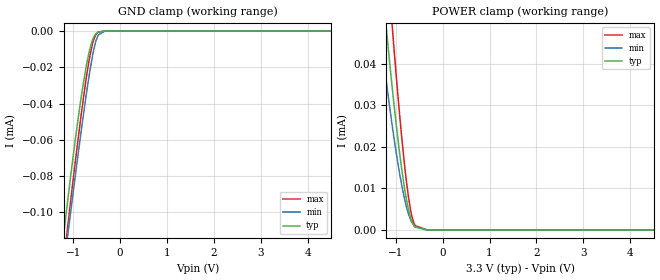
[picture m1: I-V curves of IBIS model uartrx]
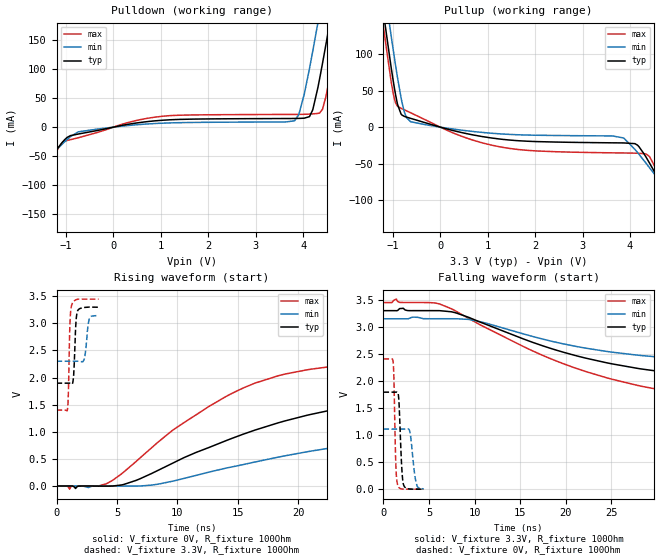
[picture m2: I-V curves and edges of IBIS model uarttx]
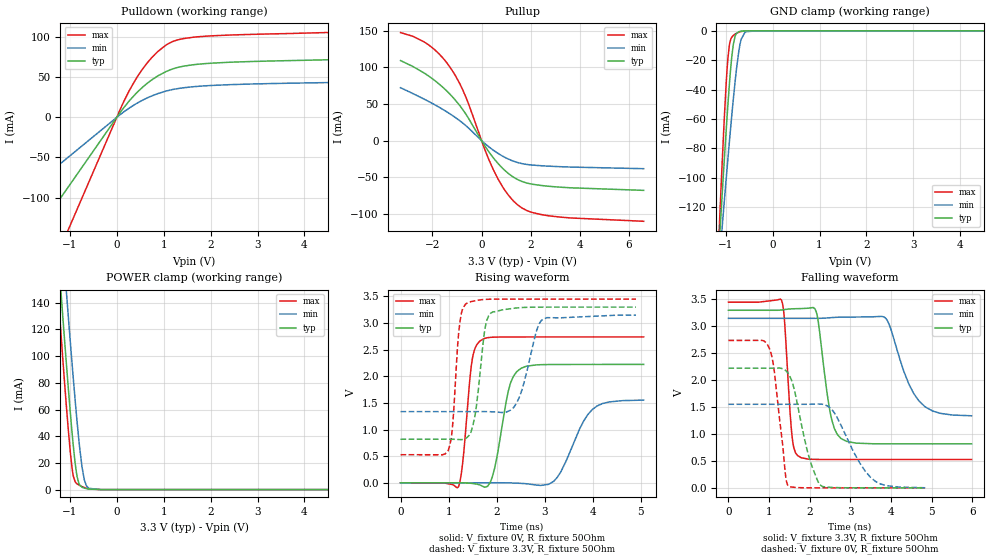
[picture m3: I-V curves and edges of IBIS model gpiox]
|Texas Instruments Incorporated
| NA
| Marketing part#   Digital Voltage Range   Package-type   #pins
| TPS65982ZQZ   3.15V-3.45V   BGA   96
[IBIS Ver]   4.1
[File name]   tps65982.ibs
[File Rev]   1.1
[Date]   8/31/2016
[Source]
| Texas Instruments Incorporated.
| Analog-eLab Design Center, HPA
| 12500 TI Blvd
| Dallas, TX -75243
[Notes]   Revision History:
| Rev 1.1: 8/31/2016
| - HRESET pin model added
| Rev 1.0: 5/5/2015
| - Initial version of the model
| - Model generated from simulations in TISPICE
| - Model matched to SPICE simulation
| - C_comp although listed in numerical order of value are
|   obtained from varying PVT conditions. For PVT conditions for
|   each specific value refer the buffer description under
|   respective [Model]. IBIS model user is responsible for using
|   appropriate C_comp to simulate for Signal Integrity.
[Disclaimer]
| This model is designed as an aid for customers of Texas Instruments.
| TI and its licensors and suppliers make no warranties, either expressed
| or implied, with respect to this  model, including the warranties of
| merchantability or fitness for a particular purpose. The model is
| provided solely on an "as is" basis. The entire risk as to its quality
| and performance is with the customer.
[Copyright]
(C) Copyright 2015 Texas Instruments Incorporated.All rights reserved.
|   TPS65982ZQZ
[Component]   TPS65982ZQZ
[Manufacturer]   TI
[Package]   |96 BGA  -  ZQZ package
|   typ   min   max
R_pkg   0.075   0.050   0.207
L_pkg   9.56E-10   6.42E-10   2.82E-09
C_pkg   0.201p   0.076p   0.723p
[Pin]  signal_name   model_name   R_pin   L_pin   C_pin
A1   GND   gnd   0.0501   6.99E-10   0.076p
A2   LDO_1V8D   power   0.0551   6.42E-10   0.199p
A3   SPI_CLK   gpiox   0.0630   7.47E-10   0.156p
A4   SPI_MISO   gpiox   0.0611   6.96E-10   0.149p
A5   I2C_SDA2   sda   0.0623   7.17E-10   0.159p
A6   PP_HV   power   0.0600   7.26E-10   0.287p
A7   PP_HV   power   0.0633   7.40E-10   0.287p
A8   PP_HV   power   0.0598   7.10E-10   0.287p
A9   HV_GATE2   nc   0.0723   8.83E-10   0.158p
A10   SENSEN   nc   0.0637   7.41E-10   0.133p
A11   PP_5V0   power   0.0647   7.77E-10   0.177p
B1   VDDIO   power   0.0565   6.69E-10   0.213p
B2   GPIO0   gpiols   0.0912   1.08E-09   0.567p
B3   SPI_SSZ   gpiox   0.0887   1.07E-09   0.247p
B4   SPI_MOSI   gpiox   0.0871   1.07E-09   0.197p
B5   I2C_SCL2   scl   0.0873   1.04E-09   0.214p
B6   I2C_IRQ2Z   od   0.1081   1.29E-09   0.251p
B7   PP_HV   power   0.0627   7.36E-10   0.287p
B8   GND   gnd   0.0594   7.56E-10   0.076p
B9   HV_GATE1   nc   0.0958   1.21E-09   0.212p
B10   SENSEP   nc   0.0955   1.20E-09   0.205p
B11   PP_5V0   power   0.0630   7.60E-10   0.357p
C1   I2C_IRQ1Z   od   0.0610   6.91E-10   0.153p
C2   GPIO1   gpiols   0.0912   1.08E-09   0.205p
C10   GPIO4   gpiols   0.0577   6.83E-10   0.149p
C11   PP_5V0   power   0.0640   7.78E-10   0.222p
D1   I2C_SDA1   sda   0.0611   6.99E-10   0.145p
D2   I2C_SCL1   scl   0.0866   1.03E-09   0.186p
D5   DEBUG_CTL2   gpiols_i2c   0.1437   1.99E-09   0.399p
D6   HRESET   hreset   0.1095   1.68E-09   0.076p
D7   GPIO7   gpiols   0.0881   1.04E-09   0.234p
D8   GND   gnd   0.1095   1.68E-09   0.076p
D10   GPIO2   gpiols   0.0866   1.02E-09   0.234p
D11   PP_5V0   power   0.0633   7.51E-10   0.357p
E1   LDO_BMC   power   0.0564   6.69E-10   0.137p
E2   UART_TX   uarttx   0.0871   1.04E-09   0.202p
E4   DEBUG_CTL1   gpiols_i2c   0.1437   1.99E-09   0.351p
E5   GND   gnd   0.0594   7.56E-10   0.076p
E6   GND   gnd   0.0594   7.56E-10   0.076p
E7   GND   gnd   0.0594   7.56E-10   0.076p
E8   GND   gnd   0.0594   7.56E-10   0.076p
E10   GPIO5   gpiols   0.1048   1.29E-09   0.253p
E11   MRESET   gpiols   0.0576   6.90E-10   0.158p
F1   I2C_ADDR   nc   0.0611   6.93E-10   0.153p
F2   UART_RX   uartrx   0.0871   1.03E-09   0.219p
F4   SWD_DATA   gpiox   0.1319   1.79E-09   0.347p
F5   GND   gnd   0.0594   7.56E-10   0.076p
F6   GND   gnd   0.0594   7.56E-10   0.076p
F7   GND   gnd   0.0594   7.56E-10   0.076p
F8   GND   gnd   0.0594   7.56E-10   0.076p
F10   BUSPOWERZ   gpiols   0.0584   7.12E-10   0.199p
F11   RESETZ   gpiols   0.0584   7.12E-10   0.186p
G1   LDO_3V3   power   0.0564   6.69E-10   0.151p
G2   R_OSC   nc   0.0563   6.67E-10   0.149p
G4   SWD_CLK   gpiox   0.1315   1.81E-09   0.337p
G5   GND   gnd   0.0594   7.56E-10   0.076p
G6   GND   gnd   0.0594   7.56E-10   0.076p
G7   GND   gnd   0.0594   7.56E-10   0.076p
G8   GND   gnd   0.0594   7.56E-10   0.076p
G10   GPIO6   gpiols   0.0870   1.06E-09   0.206p
G11   GPIO3   gpiols   0.0895   1.10E-09   0.212p
H1   VIN_3V3   power   0.0558   6.58E-10   0.164p
H2   VOUT_3V3   power   0.0663   9.10E-10   0.206p
H4   GND   gnd   0.0594   7.56E-10   0.076p
H5   GND   gnd   0.0594   7.56E-10   0.076p
H6   GPIO8   gpiols   0.2066   2.82E-09   0.452p
H7   SS   nc   0.0851   1.67E-09   0.201p
H8   GND   gnd   0.0594   7.56E-10   0.076p
H10   PP_CABLE   power   0.0851   1.67E-09   0.394p
H11   VBUS   power   0.0614   7.25E-10   0.393p
J1   AUX_P   nc   0.0866   1.03E-09   0.723p
J2   AUX_N   nc   0.0866   1.03E-09   0.723p
J10   VBUS   power   0.0618   7.45E-10   0.152p
J11   VBUS   power   0.0622   7.40E-10   0.152p
K1   LDO_1V8A   power   0.0563   6.69E-10   0.152p
K2   DEBUG2   nc   0.0616   7.07E-10   0.133p
K3   DEBUG4   nc   0.0893   1.04E-09   0.202p
K4   LSX_P2R   uarttx   0.0669   9.83E-10   0.202p
K5   USB_RP_N   nc   0.0772   1.12E-09   0.214p
K6   C_USB_TP   nc   0.0748   1.09E-09   0.200p
K7   C_USB_BP   nc   0.0776   1.14E-09   0.217p
K8   C_SBU1   nc   0.0976   1.24E-09   0.252p
K9   RPD_G1   nc   0.0899   1.09E-09   0.244p
K10   RPD_G2   nc   0.0710   1.04E-09   0.221p
K11   VBUS   power   0.0604   7.03E-10   0.076p
L1   GND   gnd   0.0594   7.56E-10   0.076p
L2   DEBUG1   nc   0.0616   7.07E-10   0.178p
L3   DEBUG3   nc   0.0893   1.04E-09   0.256p
L4   LSX_R2P   uartrx   0.0587   7.15E-10   0.148p
L5   USB_RP_P   nc   0.0701   8.92E-10   0.155p
L6   C_USB_TN   nc   0.0663   8.25E-10   0.158p
L7   C_USB_BN   nc   0.0687   8.83E-10   0.184p
L8   C_SBU2   nc   0.0748   1.09E-09   0.201p
L9   C_CC1   nc   0.0578   7.16E-10   0.207p
L10   C_CC2   nc   0.0599   7.33E-10   0.209p
L11   NC   nc   0.0976   1.24E-09   0.076p
| Models and submodels in the file (9): uartrx (Input), uarttx (Output), gpiox (I/O), gpiols (I/O), gpiols_i2c (I/O), sda (I/O_open_drain), scl (I/O_open_drain), od (Open_sink), hreset (Input)
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|   uartrx Model
[Model]   uartrx
Model_type   Input
Vinl = 0.80
Vinh = 2.00
|   typ   min   max
|   (nom PVT)   (fast PVT)   (slow PVT)
C_comp   1.884e-13   1.883e-13   1.922e-13
| Where nom  PVT is Nominal Process, 3.3V, 27C
|   Fast PVT is Strong Process,  3.45V, -40C
|   Slow PVT is Weak Process,   3.15V, 125C
[Voltage Range]   3.3   3.15   3.45
|Junction Temperature
[Temperature Range]   27   125   -40
[Power Clamp Reference]   3.3   3.15   3.45
[GND Clamp Reference]   0   0   0
[GND Clamp]
|   Voltage   I(typ)   I(min)   I(max)
-3.3V     -616.4uA   -586.9uA   -673.7uA
-1.268V   -126.8uA   -144.3uA   -142.4uA
-1.14V    -98.51uA   -117.6uA   -113uA
-1.033V   -75.66uA   -95.54uA   -89.02uA
-843.6mV  -38.94uA   -57.88uA   -48.92uA
-733.2mV  -21.02uA   -37.2uA    -27.92uA
-650.1mV  -10.41uA   -22.91uA   -14.51uA
-587.4mV  -4.818uA   -13.5uA    -6.861uA
-524.7mV  -1.682uA   -6.189uA   -2.313uA
-465mV    -476nA     -2.11uA    -584.1nA
-222.5mV  0A         0A         0A
6.6V      0A         0A         0A
[POWER Clamp]
|   Voltage   I(typ)   I(min)   I(max)
-3.3V     363.5uA    282.4uA    459.4uA
-1.331V   64.51uA    47.82uA    88.59uA
-1.206V   49.19uA    36.28uA    68.73uA
-1.122V   39.53uA    29.05uA    56.03uA
-1.061V   32.84uA    24.08uA    47.16uA
-906mV    17.59uA    12.89uA    26.45uA
-795.3mV  8.89uA     6.653uA    13.99uA
-729.8mV  5.015uA    3.913uA    8.085uA
-686.4mV  3.106uA    2.555uA    5.017uA
-588.3mV  737.6nA    762.5nA    1.066uA
-330mV    0A         11.44nA    0A
6.6V      0A         0A         0A
|   uarttx Model
[Model]   uarttx
Model_type   Output
Polarity   Non-Inverting
Vmeas = 1.65
Vref = 0
Cref = 2pF
Rref = 200
|   typ   min   max
|   (nom PVT)   (fast PVT)   (slow PVT)
C_comp   5.219e-13   4.960e-13   5.699e-13
| Where nom  PVT is Nominal Process, 3.3V, 27C
|   Fast PVT is Strong Process,  3.45V, -40C
|   Slow PVT is Weak Process,   3.15V, 125C
[Voltage Range]   3.3   3.15   3.45
|Junction Temperature
[Temperature Range]   27   125   -40
[Pullup Reference]   3.3   3.15   3.45
[Pulldown Reference]   0   0   0
[Power Clamp Reference]   3.3   3.15   3.45
[GND Clamp Reference]   0   0   0
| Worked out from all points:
|   slope of the pulldown table from 0 to 0.495 V, typ, clamps not added: 68.4 ohm
|   slope of the pullup table from 0 to 0.495 V, typ, clamps not added: 61.3 ohm
|   falling waveform, V_fixture 3.3V, R_fixture 100Ohm: 20-80 % time 18.5ns typ, 15.1ns min, 20.5ns max; typ from 3.3 V to 1.9 V
|   rising waveform, V_fixture 0V, R_fixture 100Ohm: 20-80 % time 14.5ns typ, 17.7ns min, 10.1ns max; typ from 0 V to 1.79 V
|   rising waveform, V_fixture 3.3V, R_fixture 100Ohm: 20-80 % time 158ps typ, 228ps min, 128ps max; typ from 1.9 V to 3.3 V
|   falling waveform, V_fixture 0V, R_fixture 100Ohm: 20-80 % time 271ps typ, 426ps min, 190ps max; typ from 1.79 V to 0.001 V
[Pulldown]
|   Voltage   I(typ)   I(min)   I(max)
-3.3V     -295.9mA   -222.5mA   -395.2mA
-1.723V   -100.8mA   -83.38mA   -125.5mA
-1.155V   -34.06mA   -35.23mA   -34.78mA
-742.2mV  -11.87mA   -8.083mA   -18.25mA
1.053V    11.95mA    6.868mA    18.86mA
3.819V    14.88mA    10.9mA     21.89mA
4.134V    18.24mA    101.1mA    22.45mA
4.31V     67.66mA    179mA      23.58mA
4.559V    178.9mA    295.7mA    85.55mA
4.683V    237.9mA    355.2mA    142.3mA
5.019V    401.4mA    518.3mA    305.3mA
6.6V      1.193A     1.302A     1.105A
[Pullup]
|   Voltage   I(typ)   I(min)   I(max)
-3.3V     1.215A     1.243A     1.21A
-1.216V   164.2mA    207.6mA    144.4mA
-1.037V   81.83mA    125.1mA    62.46mA
-943.8mV  44.61mA    84.81mA    33.37mA
-761.1mV  14.82mA    21.36mA    23.8mA
-625.7mV  12.02mA    7.365mA    19.69mA
1.251V    -16.27mA   -9.155mA   -26.91mA
3.866V    -21.63mA   -14.87mA   -35.39mA
4.156V    -24.62mA   -34.6mA    -35.75mA
4.411V    -49.17mA   -55.61mA   -40.34mA
5.087V    -130.2mA   -114.2mA   -146.2mA
6.6V      -317.9mA   -248.2mA   -405.3mA
[Ramp]
R_load = 100
|   typ   min   max
dV/dt_r   1.07582/1.45421e-08   0.66599/1.79204e-08   1.44461/1.00345e-08
dV/dt_f   0.841274/1.8421e-08   0.509094/1.51105e-08   1.22678/2.04399e-08
[Falling Waveform]
V_fixture = 3.3V
V_fixture_min = 3.15V
V_fixture_max = 3.45V
R_fixture = 100Ohm
|   Time   V(typ)   V(min)   V(max)
0s        3.3V       3.15V      3.45V
1.422ns   3.3V       3.15V      3.514V
1.766ns   3.336V     3.15V      3.453V
6.178ns   3.3V       3.151V     3.423V
10.67ns   3.084V     3.093V     3.032V
21.09ns   2.469V     2.64V      2.236V
27.88ns   2.233V     2.477V     1.918V
35.79ns   2.076V     2.382V     1.696V
57.46ns   1.929V     2.311V     1.47V
100ns     1.898V     2.302V     1.405V
[Rising Waveform]
V_fixture = 0V
V_fixture_min = 0V
V_fixture_max = 0V
R_fixture = 100Ohm
|   Time   V(typ)   V(min)   V(max)
0s        1.779nV    51.61nV    941pV
1.08ns    39.41uV    50.68nV    -58.51mV
4.122ns   -2.492mV   -38.34uV   41.13mV
8.372ns   285.5mV    32.82mV    804.4mV
14.01ns   834.7mV    329.1mV    1.649V
16.42ns   1.031V     442.7mV    1.898V
21.06ns   1.322V     643.8mV    2.155V
26.85ns   1.542V     821.9mV    2.282V
36.28ns   1.694V     980.9mV    2.36V
71.83ns   1.789V     1.104V     2.406V
[Rising Waveform]
V_fixture = 3.3V
V_fixture_min = 3.15V
V_fixture_max = 3.45V
R_fixture = 100Ohm
|   Time   V(typ)   V(min)   V(max)
0s        1.897V     2.301V     1.401V
900ps     1.897V     2.301V     1.406V
974ps     1.897V     2.301V     1.674V
1.128ns   1.896V     2.301V     3.084V
1.292ns   1.884V     2.301V     3.362V
1.416ns   2.041V     2.301V     3.405V
1.738ns   3.227V     2.302V     3.443V
2.308ns   3.293V     2.349V     3.446V
2.712ns   3.3V       3.083V     3.447V
3.486ns   3.297V     3.146V     3.447V
[Falling Waveform]
V_fixture = 0V
V_fixture_min = 0V
V_fixture_max = 0V
R_fixture = 100Ohm
|   Time   V(typ)   V(min)   V(max)
0s        1.794V     1.111V     2.408V
1.054ns   1.794V     1.111V     2.368V
1.148ns   1.794V     1.111V     2.067V
1.366ns   1.793V     1.111V     441.7mV
1.564ns   1.79V      1.111V     80.61mV
1.696ns   1.639V     1.111V     31.2mV
2.19ns    90.75mV    1.111V     2.688mV
2.864ns   3.776mV    1.084V     739.1uV
3.594ns   1.059mV    113.8mV    742uV
4.408ns   691.5uV    4.016mV    764uV
|   gpiox Model
[Model]   gpiox
Model_type   I/O
Polarity   Non-Inverting
Enable   Active-High
Vinl = 0.80
Vinh = 2.00
Vmeas = 1.65
Vref = 0
Cref = 2pF
Rref = 100
|   typ   min   max
|   (nom PVT)   (fast PVT)   (slow PVT)
C_comp   1.059e-12   1.036e-12   1.086e-12
| Where nom  PVT is Nominal Process, 3.3V, 27C
|   Fast PVT is Strong Process,  3.45V, -40C
|   Slow PVT is Weak Process,   3.15V, 125C
[Voltage Range]   3.3   3.15   3.45
|Junction Temperature
[Temperature Range]   27   125   -40
[Pullup Reference]   3.3   3.15   3.45
[Pulldown Reference]   0   0   0
[Power Clamp Reference]   3.3   3.15   3.45
[GND Clamp Reference]   0   0   0
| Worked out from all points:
|   slope of the pulldown table from 0 to 0.495 V, typ, clamps not added: 14.3 ohm
|   slope of the pullup table from 0 to 0.495 V, typ, clamps not added: 20.4 ohm
|   GND clamp passes 1 mA (typ) near -0.74 V on its own axis
|   POWER clamp passes 1 mA (typ) near -0.68 V on its own axis
|   falling waveform, V_fixture 3.3V, R_fixture 50Ohm: 20-80 % time 269ps typ, 546ps min, 145ps max; typ from 3.3 V to 0.818 V
|   rising waveform, V_fixture 0V, R_fixture 50Ohm: 20-80 % time 262ps typ, 477ps min, 159ps max; typ from 0 V to 2.22 V
|   rising waveform, V_fixture 3.3V, R_fixture 50Ohm: 20-80 % time 184ps typ, 301ps min, 129ps max; typ from 0.818 V to 3.3 V
|   falling waveform, V_fixture 0V, R_fixture 50Ohm: 20-80 % time 402ps typ, 647ps min, 241ps max; typ from 2.22 V to 0 V
[Pulldown]
|   Voltage   I(typ)   I(min)   I(max)
-3.3V     -277mA     -158.5mA   -447.7mA
-150.2mV  -12.61mA   -7.21mA    -20.37mA
151.8mV   12.28mA    6.938mA    20.02mA
274.2mV   21.1mA     11.96mA    34.21mA
460.5mV   32.75mA    18.65mA    52.7mA
653.4mV   42.71mA    24.42mA    68.26mA
854.7mV   51.01mA    29.25mA    81.01mA
1.178V    60.18mA    34.6mA     94.27mA
1.422V    63.9mA     36.96mA    98.32mA
2.041V    67.72mA    39.9mA     101.8mA
5.432V    73.05mA    44.32mA    107.3mA
6.6V      76.33mA    46.37mA    112.1mA
[GND Clamp]
|   Voltage   I(typ)   I(min)   I(max)
-3.3V     -1.417A    -1.066A    -1.893A
-1.199V   -179.2mA   -182.9mA   -181.3mA
-1.116V   -133.7mA   -150mA     -119.5mA
-1.076V   -112.1mA   -134.2mA   -90.78mA
-988.5mV  -67.46mA   -100.7mA   -35.54mA
-953.7mV  -50.94mA   -87.68mA   -19.31mA
-909.2mV  -31.72mA   -71.45mA   -7.69mA
-838.2mV  -9.42mA    -46.98mA   -3.178mA
-720.1mV  -595uA     -13.97mA   -982.8uA
-581.6mV  -40.13uA   -626.1uA   -81.68uA
-330mV    -70.13nA   -605.5nA   -45.49nA
6.6V      0A         0A         0A
[Pullup]
|   Voltage   I(typ)   I(min)   I(max)
-3.3V     109.3mA    72.2mA     147.5mA
-2.134V   87.66mA    53.06mA    130.1mA
-1.567V   72.53mA    42.38mA    112.5mA
-1.216V   60.85mA    34.92mA    96.78mA
-626.2mV  35.49mA    20.06mA    58.32mA
146.6mV   -7.842mA   -4.352mA   -13.36mA
521.4mV   -25.32mA   -14.14mA   -42.61mA
1.053V    -43.8mA    -24.62mA   -72.71mA
1.475V    -53.28mA   -29.99mA   -87.89mA
2.005V    -59.17mA   -33.21mA   -97.51mA
2.831V    -62.63mA   -35.06mA   -103.1mA
6.6V      -67.93mA   -38.33mA   -110.2mA
[POWER Clamp]
|   Voltage   I(typ)   I(min)   I(max)
-3.3V     1.237A     1.263A     1.239A
-1.258V   181mA      234.5mA    150.2mA
-1.144V   126.7mA    180.8mA    94.91mA
-1.076V   95.5mA     149.5mA    63.67mA
-1.033V   76.43mA    130.1mA    45.13mA
-990mV    57.86mA    110.8mA    28.14mA
-930.6mV  34.46mA    85.16mA    11.11mA
-844.8mV  9.689mA    50.62mA    4.235mA
-739mV    1.755mA    16.64mA    2.217mA
-647mV    743.2uA    2.889mA    1.001mA
-330mV    1.406uA    4.138uA    685.6nA
6.6V      0A         0A         0A
[Ramp]
R_load = 50
|   typ   min   max
dV/dt_r   1.33389/2.60015e-10   0.931714/4.70432e-10   1.64372/1.58172e-10
dV/dt_f   1.48927/2.68363e-10   1.08801/5.43452e-10   1.75377/1.45042e-10
[Falling Waveform]
V_fixture = 3.3V
V_fixture_min = 3.15V
V_fixture_max = 3.45V
R_fixture = 50Ohm
|   Time   V(typ)   V(min)   V(max)
0s        3.3V       3.15V      3.45V
1.306ns   3.305V     3.15V      3.488V
1.56ns    3.326V     3.15V      997mV
1.7ns     3.329V     3.15V      600.9mV
2.16ns    3.271V     3.149V     528.9mV
2.51ns    1.375V     3.162V     527.5mV
2.776ns   913.8mV    3.172V     527.2mV
3.83ns    818.6mV    3.175V     527.1mV
4.68ns    817.9mV    1.622V     527.1mV
5.982ns   817.9mV    1.339V     527.1mV
[Rising Waveform]
V_fixture = 0V
V_fixture_min = 0V
V_fixture_max = 0V
R_fixture = 50Ohm
|   Time   V(typ)   V(min)   V(max)
0s        505.5pV    14.97nV    196.3pV
1.202ns   574.3uV    426.7nV    -79.46mV
1.494ns   -12.58mV   -3.585uV   2.327V
1.654ns   -41.27mV   -26.69uV   2.667V
1.886ns   49.79mV    228.1uV    2.733V
2.242ns   1.722V     -1.633mV   2.739V
2.508ns   2.151V     -11.3mV    2.739V
3.186ns   2.222V     27.84mV    2.74V
4.09ns    2.223V     1.444V     2.74V
5.058ns   2.223V     1.553V     2.74V
[Rising Waveform]
V_fixture = 3.3V
V_fixture_min = 3.15V
V_fixture_max = 3.45V
R_fixture = 50Ohm
|   Time   V(typ)   V(min)   V(max)
0s        817.9mV    1.337V     527mV
988ps     818.1mV    1.337V     597.7mV
1.078ns   817.6mV    1.337V     1.024V
1.236ns   811.5mV    1.337V     3.021V
1.36ns    832.2mV    1.337V     3.362V
1.55ns    1.265V     1.337V     3.419V
1.874ns   3.184V     1.335V     3.448V
2.426ns   3.285V     1.52V      3.45V
2.932ns   3.3V       3.052V     3.45V
4.898ns   3.3V       3.15V      3.45V
[Falling Waveform]
V_fixture = 0V
V_fixture_min = 0V
V_fixture_max = 0V
R_fixture = 50Ohm
|   Time   V(typ)   V(min)   V(max)
0s        2.223V     1.553V     2.74V
1.002ns   2.223V     1.553V     2.599V
1.104ns   2.224V     1.553V     2.299V
1.394ns   2.189V     1.553V     301.3mV
1.472ns   2.124V     1.553V     36.68mV
2.002ns   520.6mV    1.554V     770.1uV
2.25ns    57.55mV    1.557V     204.5uV
2.606ns   6.093mV    1.393V     39.09uV
3.616ns   37.19uV    119.7mV    1.922uV
4.838ns   1.764uV    1.853mV    717.1nV
